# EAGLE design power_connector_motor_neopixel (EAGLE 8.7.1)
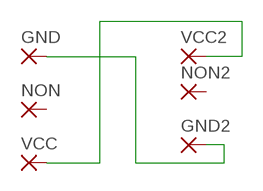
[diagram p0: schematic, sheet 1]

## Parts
GND  SMD2  [SMD1,27-2,54]
GND2  SMD2  [SMD1,27-2,54]
NON  SMD2  [SMD1,27-2,54]
NON2  SMD2  [SMD1,27-2,54]
VCC  SMD2  [SMD1,27-2,54]
VCC2  SMD2  [SMD1,27-2,54]

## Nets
N$1: GND2.1(P) GND.1(P)
N$3: VCC2.1(P) VCC.1(P)
Unconnected: NON2.1(P) NON.1(P)

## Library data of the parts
GND GND2 NON NON2 VCC VCC2 = wirepad:SMD2: SMD PAD

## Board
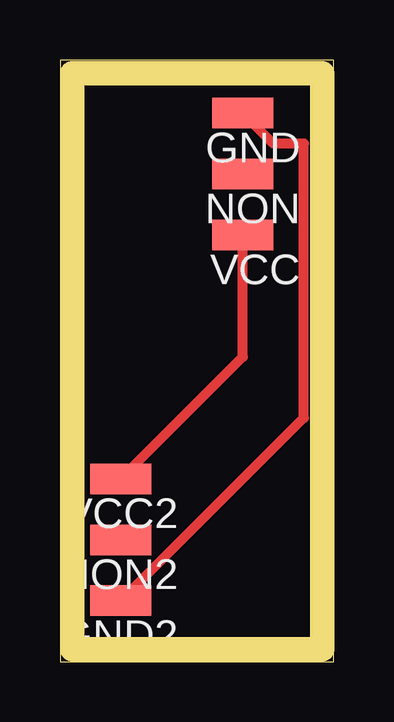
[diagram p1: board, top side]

Size 11.41 x 25.07 mm. Coordinates in mm from the lower left corner, seen from the top.
Outline: 0,0 11.41,0 11.41,25.07 0,25.07 0,0
Copper layers (1*16): Top 0.035mm / dielectric 1.5mm / Bottom 0.035mm
Design rules "default": minimum track width 6mil, minimum drill 0.35mm, track to track 6mil, track to pad 6mil, pad to pad 6mil, via to via 6mil, smd to smd 6mil, copper to edge 40mil, drill to drill 6mil, minimum pad ring 10mil, minimum via ring 8mil, stop-mask expansion 4mil, vias tented up to drill 0mil, thermal gap 10mil
Milling: 4 lines

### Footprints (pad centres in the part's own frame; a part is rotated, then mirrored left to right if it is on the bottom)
SMD1,27-2,54 = smd 1.27 x 2.54: 1 0,0

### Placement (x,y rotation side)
GND  7.62,22.86 90 top
GND2  2.54,2.54 90 top
NON  7.62,20.32 90 top
NON2  2.54,5.08 90 top
VCC  7.62,17.78 90 top
VCC2  2.54,7.62 90 top

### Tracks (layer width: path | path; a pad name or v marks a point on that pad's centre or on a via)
N$1
  Top 0.406: GND2.1 10.16,10.16 10.16,21.59 8.89,21.59 GND.1
N$3
  Top 0.406: VCC2.1 7.62,12.7 VCC.1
